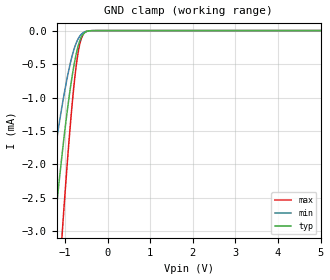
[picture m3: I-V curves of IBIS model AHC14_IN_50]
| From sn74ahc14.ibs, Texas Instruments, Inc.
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[Model]   AHC14_IN_50
Model_type  Input
Vinl=1.57
Vinh=3.57
| variable   typ   min   max
C_comp   0.55pF   0.47pF   0.65pF
[Temperature Range]   40   100   -40
| Ambient temperature   25   85   -40
[Voltage range]   5   4.5   5.5
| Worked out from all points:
|   GND clamp passes 1 mA (typ) near -0.91 V on its own axis
[GND Clamp]
| AHC14_IN_50
|   Voltage   I(typ)   I(min)   I(max)
-5V       -39.11mA   -25.82mA   -49.93mA
-1.5V     -4.697mA   -3.004mA   -7.41mA
-1.27V    -3.086mA   -1.942mA   -5.002mA
-1.245V   -2.922mA   -1.834mA   -4.75mA
-1.07V    -1.853mA   -1.127mA   -3.059mA
-1.05V    -1.74mA    -1.053mA   -2.875mA
-875mV    -857.1uA   -484.4uA   -1.403mA
-765mV    -433uA     -232.7uA   -669.5uA
-665mV    -173.1uA   -93.85uA   -234uA
-615mV    -93.6uA    -53.59uA   -114.4uA
-545mV    -32.78uA   -20.84uA   -33.45uA
5V        15.07nA    1.006nA    138.2nA
